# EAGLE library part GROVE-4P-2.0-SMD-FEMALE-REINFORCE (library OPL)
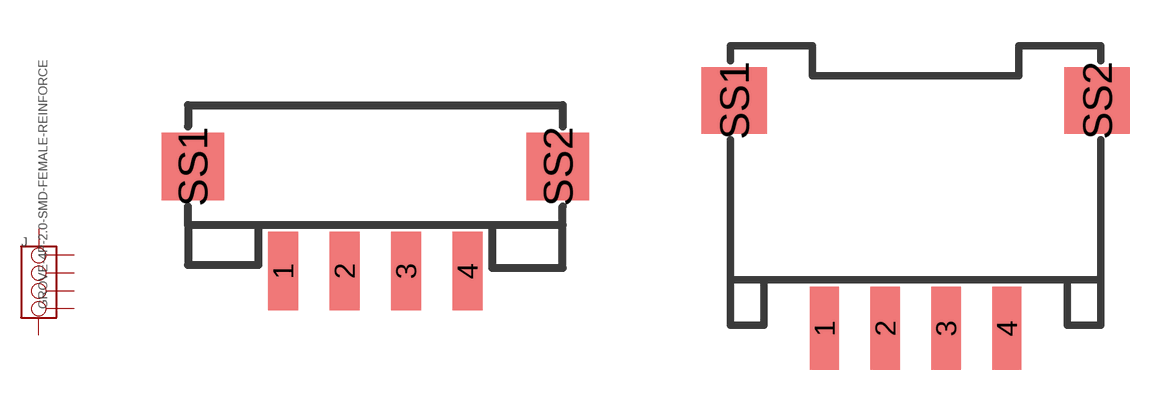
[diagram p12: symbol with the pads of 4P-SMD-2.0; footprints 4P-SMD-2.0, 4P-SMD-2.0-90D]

Designator prefix J

## GROVE-4P-2.0-SMD-FEMALE-REINFORCE-3470090P1  [4P-SMD-2.0]
1  1
2  2
3  3
4  4
SS1  SS1
SS2  SS2

## GROVE-4P-2.0-SMD-FEMALE-REINFORCE-3470120P1  [4P-SMD-2.0-90D]
Pads as for 4P-SMD-2.0

## Footprint 4P-SMD-2.0 (pad centres in mm)
3470090P1
smd 0.965 x 2.54: 1 -3,0; 2 -1,0; 3 1,0; 4 3,0
smd 2.032 x 2.184: SS1 -5.946,3.4; SS2 5.946,3.4

## Footprint 4P-SMD-2.0-90D (pad centres in mm)
3470120P1
smd 0.965 x 2.74: 1 -3,-0.1; 2 -1,-0.1; 3 1,-0.1; 4 3,-0.1
smd 2.159 x 2.184: SS1 -5.974,7.4; SS2 5.974,7.4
